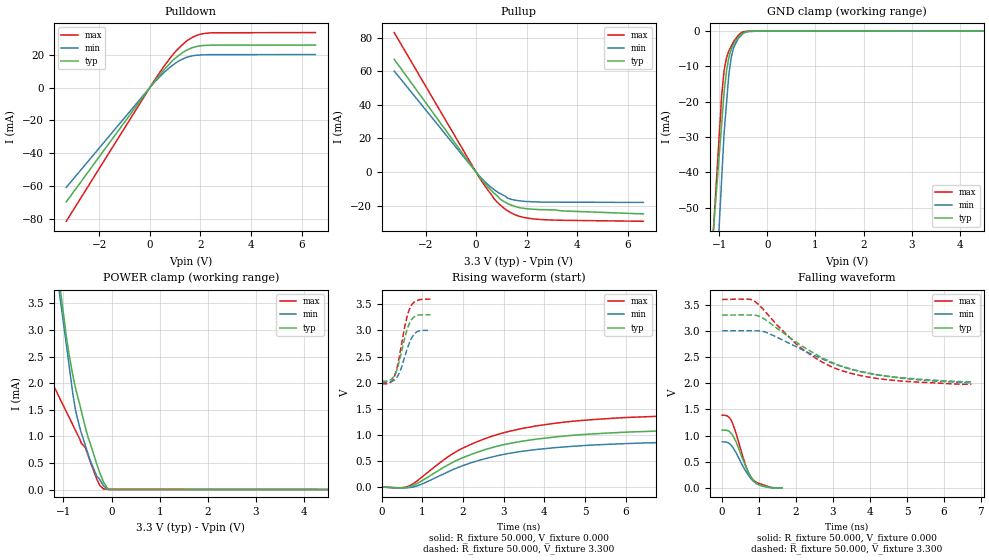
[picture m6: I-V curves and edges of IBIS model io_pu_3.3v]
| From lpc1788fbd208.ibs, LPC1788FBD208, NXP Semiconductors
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[Model]   io_pu_3.3v
Model_type I/O
Vinl=9.900E-01
Vinh=2.310E+00
Vref=0.000E+00
Rref=1.000E+06
Cref=0.000E+00
Vmeas=1.650E+00
C_comp   6.060E-13   5.760E-13   6.360E-13
[Voltage Range]   3.300E+00   3.000E+00   3.600E+00
[POWER Clamp Reference]   3.300E+00   3.000E+00   3.600E+00
[GND Clamp Reference]   0.000E+00   0.000E+00   0.000E+00
[Pullup Reference]   3.300E+00   3.000E+00   3.600E+00
[Pulldown Reference]   0.000E+00   0.000E+00   0.000E+00
[Temperature Range]   25   85   -40
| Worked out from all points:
|   slope of the pulldown table from 0 to 0.495 V, typ, clamps not added: 51.4 ohm
|   slope of the pullup table from 0 to 0.495 V, typ, clamps not added: 53.6 ohm
|   GND clamp passes 1 mA (typ) near -0.54 V on its own axis
|   POWER clamp passes 1 mA (typ) near -0.49 V on its own axis
|   rising waveform, R_fixture 50.000, V_fixture 0.000: 20-80 % time 2.29ns typ, 2.31ns min, 2.24ns max; typ from 0 V to 1.1 V
|   falling waveform, R_fixture 50.000, V_fixture 0.000: 20-80 % time 396ps typ, 429ps min, 378ps max; typ from 1.1 V to 0 V
|   rising waveform, R_fixture 50.000, V_fixture 3.300: 20-80 % time 251ps typ, 258ps min, 246ps max; typ from 2.03 V to 3.3 V
|   falling waveform, R_fixture 50.000, V_fixture 3.300: 20-80 % time 1.94ns typ, 2.12ns min, 1.72ns max; typ from 3.3 V to 2.03 V
[GND Clamp]
-3.3V     -438.5mA   -646.2mA   -539.2mA
-950mV    -26.12mA   -41.76mA   -18.22mA
-900mV    -17.35mA   -28.9mA    -11.22mA
-850mV    -11.36mA   -20.52mA   -7.6mA
-800mV    -7.442mA   -12.15mA   -5.625mA
-750mV    -5.079mA   -7.409mA   -4.294mA
-700mV    -3.596mA   -4.64mA    -2.964mA
-600mV    -1.693mA   -2.032mA   -1.181mA
-500mV    -488.5uA   -682uA     -233.7uA
-400mV    -173.2uA   -129.9uA   -101.2uA
-200mV    -62.56uA   -47.1uA    -77.07uA
6.6V      35.04uA    32.39uA    35.06uA
[Power Clamp]
-3.24V    19.03mA    18.2mA     5.713mA
-924.7mV  2.781mA    2.629mA    1.437mA
-805mV    2.145mA    1.804mA    1.216mA
-745.1mV  1.897mA    1.475mA    1.105mA
-665.3mV  1.616mA    1.183mA    959.4uA
-545.5mV  1.176mA    832.6uA    791.6uA
-445.7mV  877.7uA    553.9uA    532.7uA
-306mV    477.3uA    253.1uA    198.3uA
-246.1mV  317uA      192.2uA    82.37uA
-166.3mV  139.1uA    70.82uA    10.73uA
-66.46mV  0A         0A         10.73uA
6.6V      0A         0A         0A
[Pullup]
-3.24V    67.13mA    60.13mA    83.01mA
153.1mV   -3.115mA   -2.633mA   -3.8mA
472.4mV   -8.877mA   -7.516mA   -10.8mA
731.9mV   -12.79mA   -10.65mA   -16.25mA
951.5mV   -16mA      -12.79mA   -19.57mA
1.111V    -17.61mA   -14.02mA   -21.61mA
1.291V    -19.04mA   -15.72mA   -23.43mA
1.69V     -21.07mA   -17.04mA   -26.21mA
2.369V    -22.24mA   -17.77mA   -28.02mA
3.386V    -23.09mA   -17.92mA   -28.68mA
6.62V     -24.89mA   -18.05mA   -29.29mA
[Pulldown]
-3.3V     -69.51mA   -60.72mA   -81.36mA
173mV     3.544mA    3.051mA    4.203mA
572.2mV   11.04mA    9.362mA    13.26mA
851.6mV   15.69mA    13.04mA    18.9mA
1.151V    19.67mA    16.22mA    24.12mA
1.45V     22.74mA    18.41mA    28.3mA
1.85V     25.01mA    19.67mA    31.76mA
2.428V    25.82mA    20.06mA    33.34mA
6.54V     25.88mA    20.09mA    33.48mA
[Rising Waveform]
R_fixture = 50.000
V_fixture = 0.000
V_fixture_min = 0.000
V_fixture_max = 0.000
|  time   V(typ)   V(min)   V(max)
0s        0V         0V         -108.1uV
459.5ps   -10.85mV   -11.41mV   -10.61mV
669.2ps   7.036mV    -8.375mV   22.84mV
1.029ns   141.7mV    72.83mV    219.2mV
1.588ns   408mV      278.2mV    559mV
1.938ns   546.5mV    395.9mV    726.4mV
2.657ns   745.7mV    568.7mV    961.5mV
3.406ns   873.9mV    681.6mV    1.116V
5.324ns   1.026V     811.7mV    1.301V
8.55ns    1.103V     879.4mV    1.387V
[Falling Waveform]
R_fixture = 50.000
V_fixture = 0.000
V_fixture_min = 0.000
V_fixture_max = 0.000
|  time   V(typ)   V(min)   V(max)
0s        1.103V     879.4mV    1.387V
149.1ps   1.094V     865.2mV    1.369V
258.4ps   1.032V     802.1mV    1.269V
380ps     872.7mV    666.2mV    1.035V
636.1ps   412.4mV    322.5mV    427.7mV
805.1ps   181.7mV    154.5mV    181.4mV
920ps     95.74mV    84.37mV    109.7mV
1.07ns    45.07mV    37.54mV    67.8mV
1.34ns    4.345mV    2.922mV    7.915mV
1.62ns    0V         0V         -108.1uV
[Rising Waveform]
R_fixture = 50.000
V_fixture = 3.300
V_fixture_min = 3.000
V_fixture_max = 3.600
|  time   V(typ)   V(min)   V(max)
0s        2.028V     2.01V      1.979V
208.3ps   2.052V     2.017V     2.002V
317.4ps   2.146V     2.056V     2.13V
376.9ps   2.258V     2.108V     2.287V
440ps     2.436V     2.201V     2.528V
595.1ps   2.939V     2.572V     3.173V
654.6ps   3.083V     2.712V     3.348V
714.1ps   3.183V     2.824V     3.461V
882.7ps   3.29V      2.981V     3.577V
1.2ns     3.3V       3V         3.6V
[Falling Waveform]
R_fixture = 50.000
V_fixture = 3.300
V_fixture_min = 3.000
V_fixture_max = 3.600
|  time   V(typ)   V(min)   V(max)
0s        3.3V       3V         3.6V
848.7ps   3.299V     3V         3.579V
998.5ps   3.279V     2.998V     3.493V
1.19ns    3.204V     2.971V     3.346V
2.077ns   2.747V     2.67V      2.703V
2.686ns   2.493V     2.47V      2.41V
3.195ns   2.334V     2.326V     2.248V
3.774ns   2.221V     2.215V     2.14V
4.553ns   2.127V     2.121V     2.059V
6.74ns    2.028V     2.01V      1.979V
[Ramp]
dV/dt_r   6.6398E-01/2.2826E-09   5.2663E-01/2.2984E-09   8.3162E-01/2.2450E-09
dV/dt_f   7.6318E-01/1.9388E-09   5.9404E-01/2.1204E-09   9.7259E-01/1.7147E-09
R_load = 50
